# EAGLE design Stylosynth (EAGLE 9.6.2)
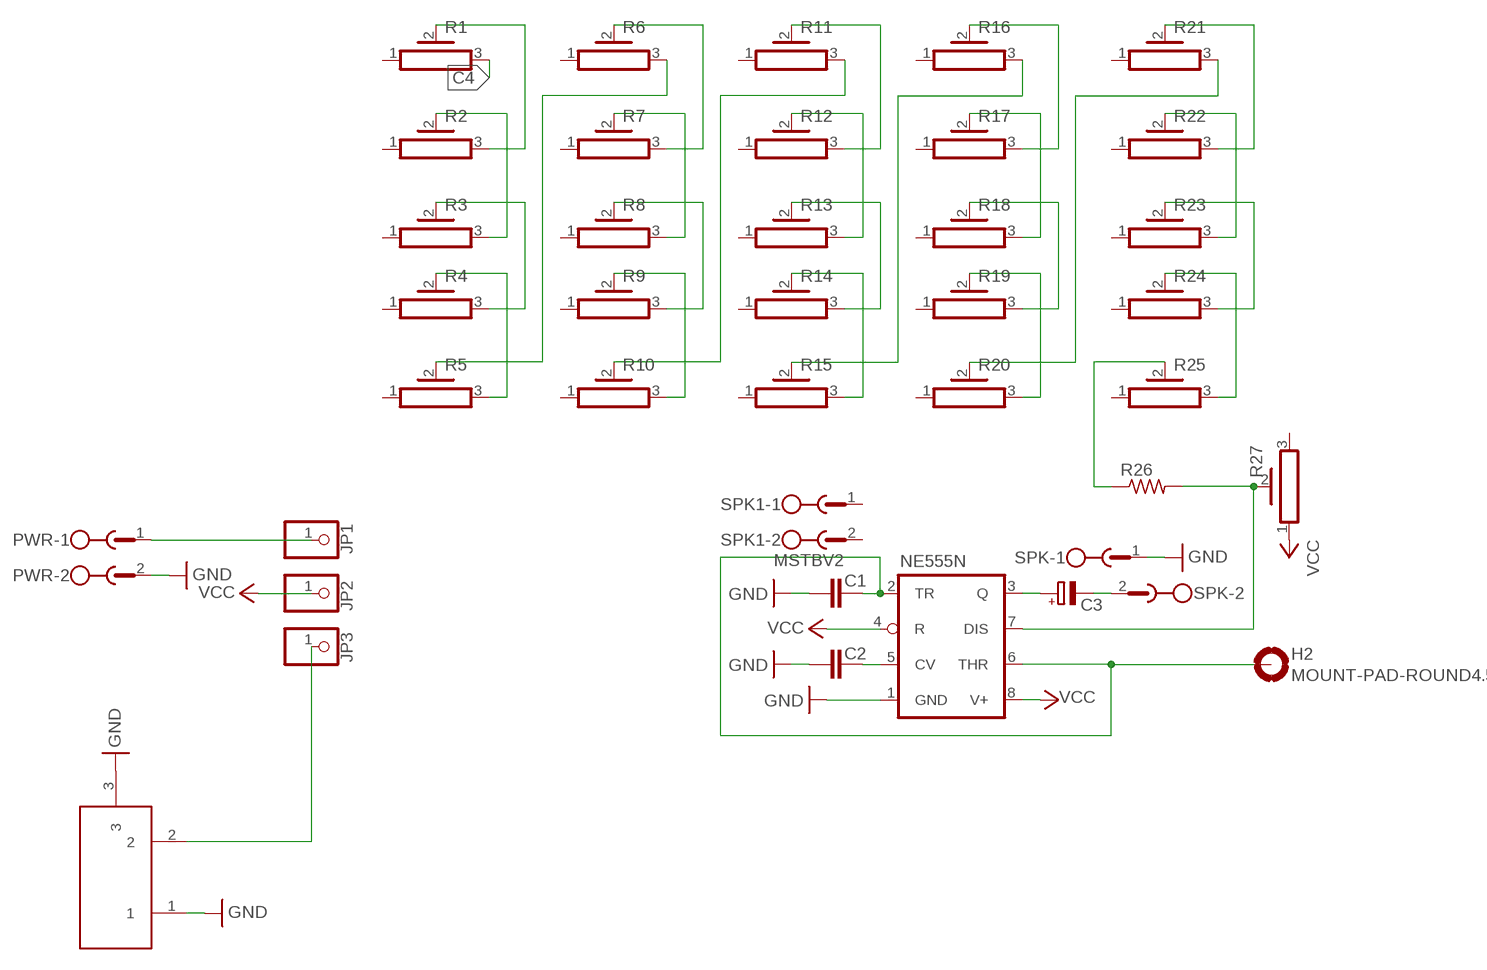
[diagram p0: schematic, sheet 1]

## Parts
C1  C5/2.5  [C5B2.5]
C2  C5/2.5  [C5B2.5]
C3  CPOL-EUE2.5-6  [E2,5-6]
H2  MOUNT-PAD-ROUND4.5  [4,5-PAD]
IC1  NE555N  [DIL08]
JP1  PINHD-1X01_2.54-90°  [1X01/90]
JP2  PINHD-1X01_2.54-90°  [1X01/90]
JP3  PINHD-1X01_2.54-90°  [1X01/90]
PWR  MSTBV2  [MSTBV2]
R1  POT_HA-06  [HA-06-SM065]
R2  POT_HA-06  [HA-06-SM065]
R3  POT_HA-06  [HA-06-SM065]
R4  POT_HA-06  [HA-06-SM065]
R5  POT_HA-06  [HA-06-SM065]
R6  POT_HA-06  [HA-06-SM065]
R7  POT_HA-06  [HA-06-SM065]
R8  POT_HA-06  [HA-06-SM065]
R9  POT_HA-06  [HA-06-SM065]
R10  POT_HA-06  [HA-06-SM065]
R11  POT_HA-06  [HA-06-SM065]
R12  POT_HA-06  [HA-06-SM065]
R13  POT_HA-06  [HA-06-SM065]
R14  POT_HA-06  [HA-06-SM065]
R15  POT_HA-06  [HA-06-SM065]
R16  POT_HA-06  [HA-06-SM065]
R17  POT_HA-06  [HA-06-SM065]
R18  POT_HA-06  [HA-06-SM065]
R19  POT_HA-06  [HA-06-SM065]
R20  POT_HA-06  [HA-06-SM065]
R21  POT_HA-06  [HA-06-SM065]
R22  POT_HA-06  [HA-06-SM065]
R23  POT_HA-06  [HA-06-SM065]
R24  POT_HA-06  [HA-06-SM065]
R25  POT_HA-06  [HA-06-SM065]
R26  R-US_0204/7  [0204/7]
R27  POT_HA-06  [HA-06-SM065]
SPK  MSTBV2  [MSTBV2]
SPK1  MSTBV2  [MSTBV2]
X1  DC21MMX  [DC-21MM]

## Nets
A4: R9.2 R10.3
A5: R21.2 R22.3
A#4: R10.2 R11.3
A#5: R22.2 R23.3
B4: R11.2 R12.3
B5: R23.2 R24.3
C4: R1.3
C5: R12.2 R13.3
C6: R24.2 R25.3
C#4: R1.2 R2.3
C#5: R13.2 R14.3
D4: R2.2 R3.3
D5: R14.2 R15.3
D#4: R3.2 R4.3
D#5: R15.2 R16.3
E4: R4.2 R5.3
E5: R16.2 R17.3
F4: R5.2 R6.3
F5: R17.2 R18.3
F#4: R6.2 R7.3
F#5: R18.2 R19.3
G4: R7.2 R8.3
G5: R19.2 R20.3
G#4: R8.2 R9.3
G#5: R20.2 R21.3
GND: C1.1 C2.1 IC1.1(GND) PWR.2 SPK.1 X1.1 X1.3
N$4: JP1.1 PWR.1
N$28: R25.2 R26.1
N$29: IC1.7(DIS) R26.2 R27.2
N$30: C3.+ IC1.3(Q)
N$31: C3.- SPK.2
N$32: C1.2 H2.B4,5(MOUNT) IC1.2(TR) IC1.6(THR)
N$33: C2.2 IC1.5(CV)
N$34: JP3.1 X1.2
VCC: IC1.4(R) IC1.8(V+) JP2.1 R27.1
Unconnected: R1.1 R2.1 R3.1 R4.1 R5.1 R6.1 R7.1 R8.1 R9.1 R10.1 R11.1 R12.1 R13.1 R14.1 R15.1 R16.1 R17.1 R18.1 R19.1 R20.1 R21.1 R22.1 R23.1 R24.1 R25.1 R27.3 SPK1.1 SPK1.2

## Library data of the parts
C1 C2 = capacitor-wima:C: CAPACITOR
C3 = rcl:CPOL-EU: POLARIZED CAPACITOR, European symbol; SPICEPREFIX: C
H2 = holes:MOUNT-PAD-ROUND: MOUNTING PAD, round
IC1 = linear:*555: TIMER
JP1-JP3 = pinhead-2:PINHD-1X01: PIN HEADER
PWR SPK SPK1 = con-phoenix-508:MSTBV2: PHOENIX; MPN: MSTBV 2,5/2-GF-5.08; OC_FARNELL: 1792792; OC_NEWARK: 69R9845
R1-R25 R27 = Tinkercad:POT: Rectangular Trimmer Potentiometers - PV36 Series Datasheet
R26 = rcl:R-US_: RESISTOR, American symbol; SPICEPREFIX: R
X1 = powersupply:DC21MM

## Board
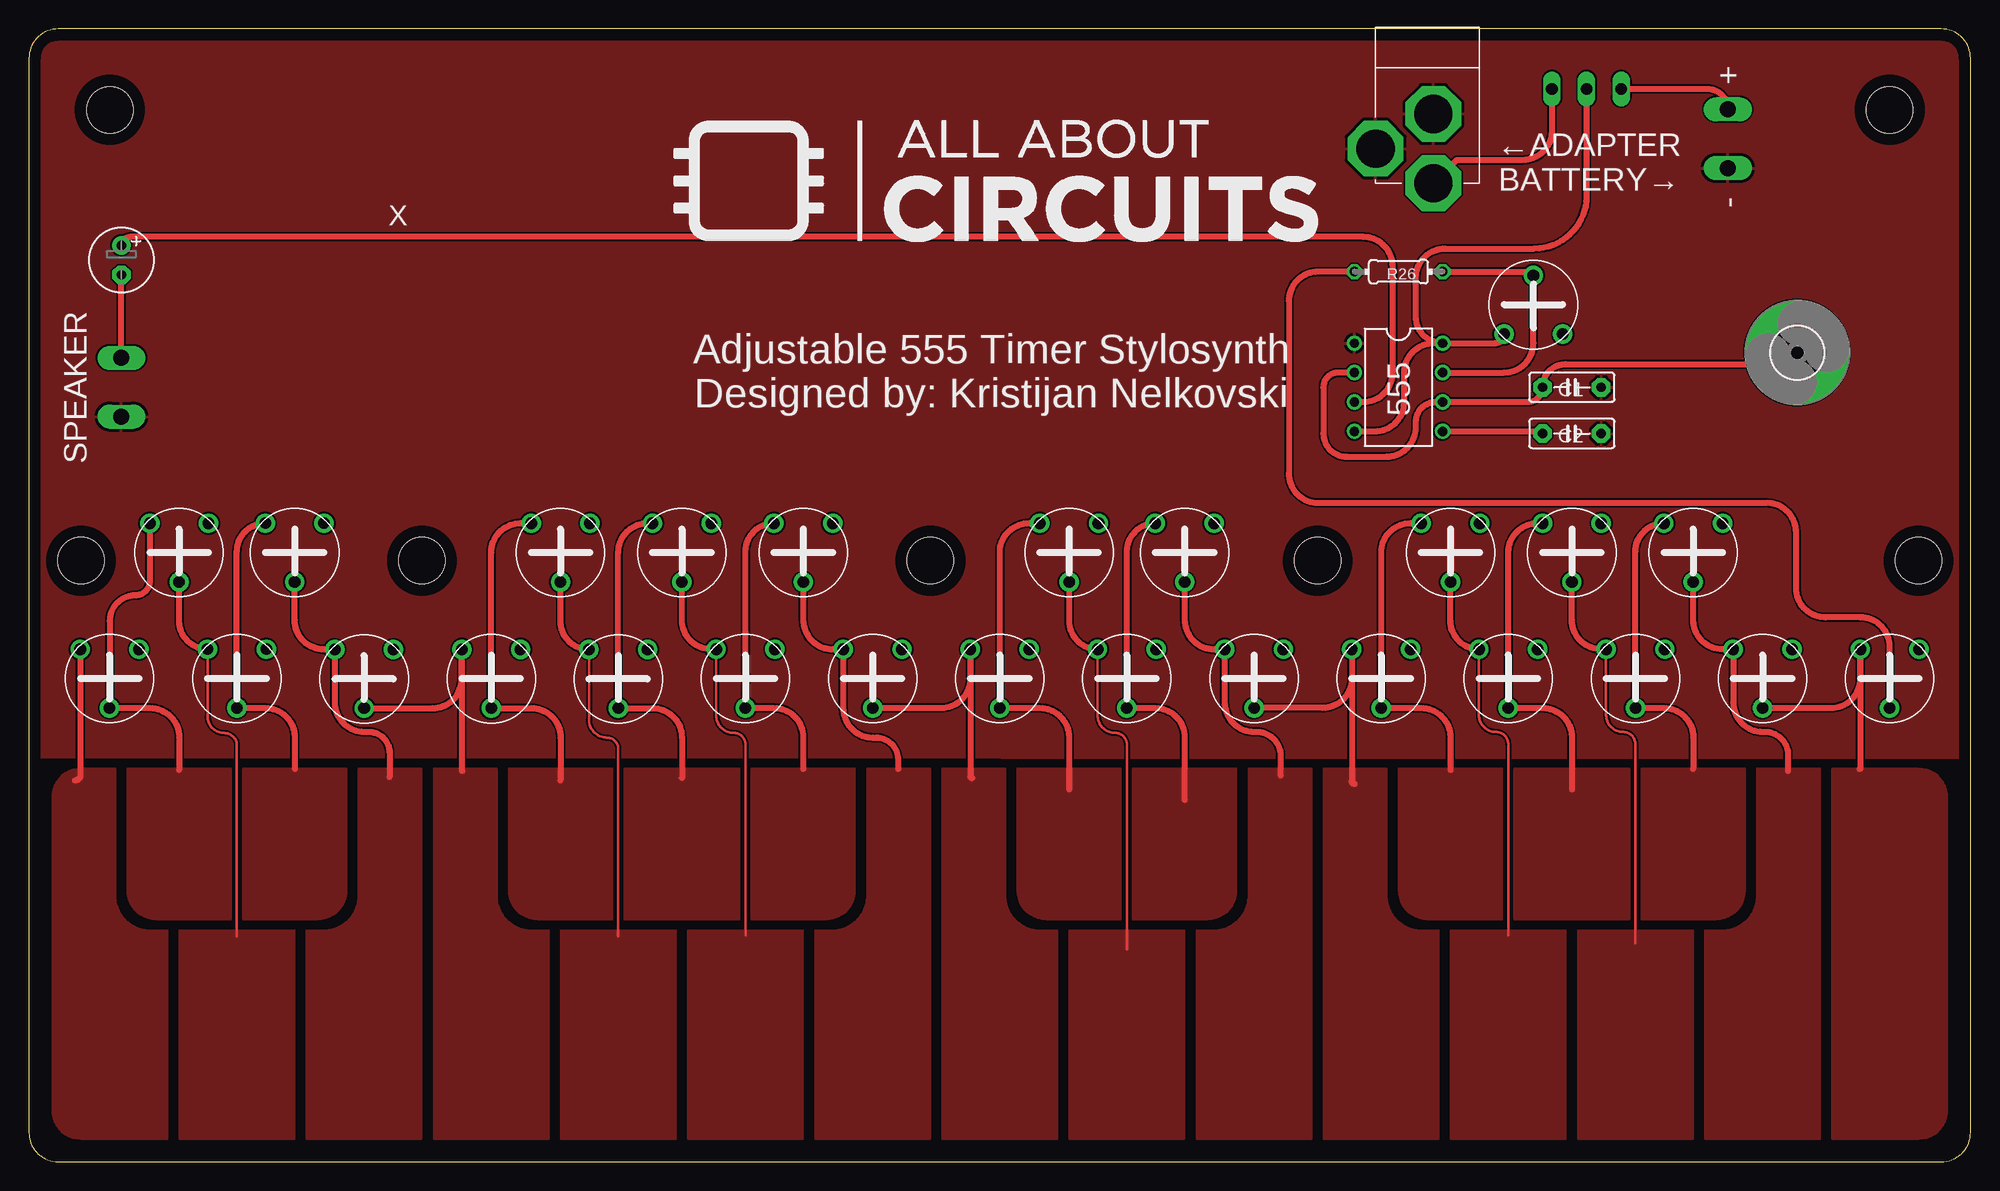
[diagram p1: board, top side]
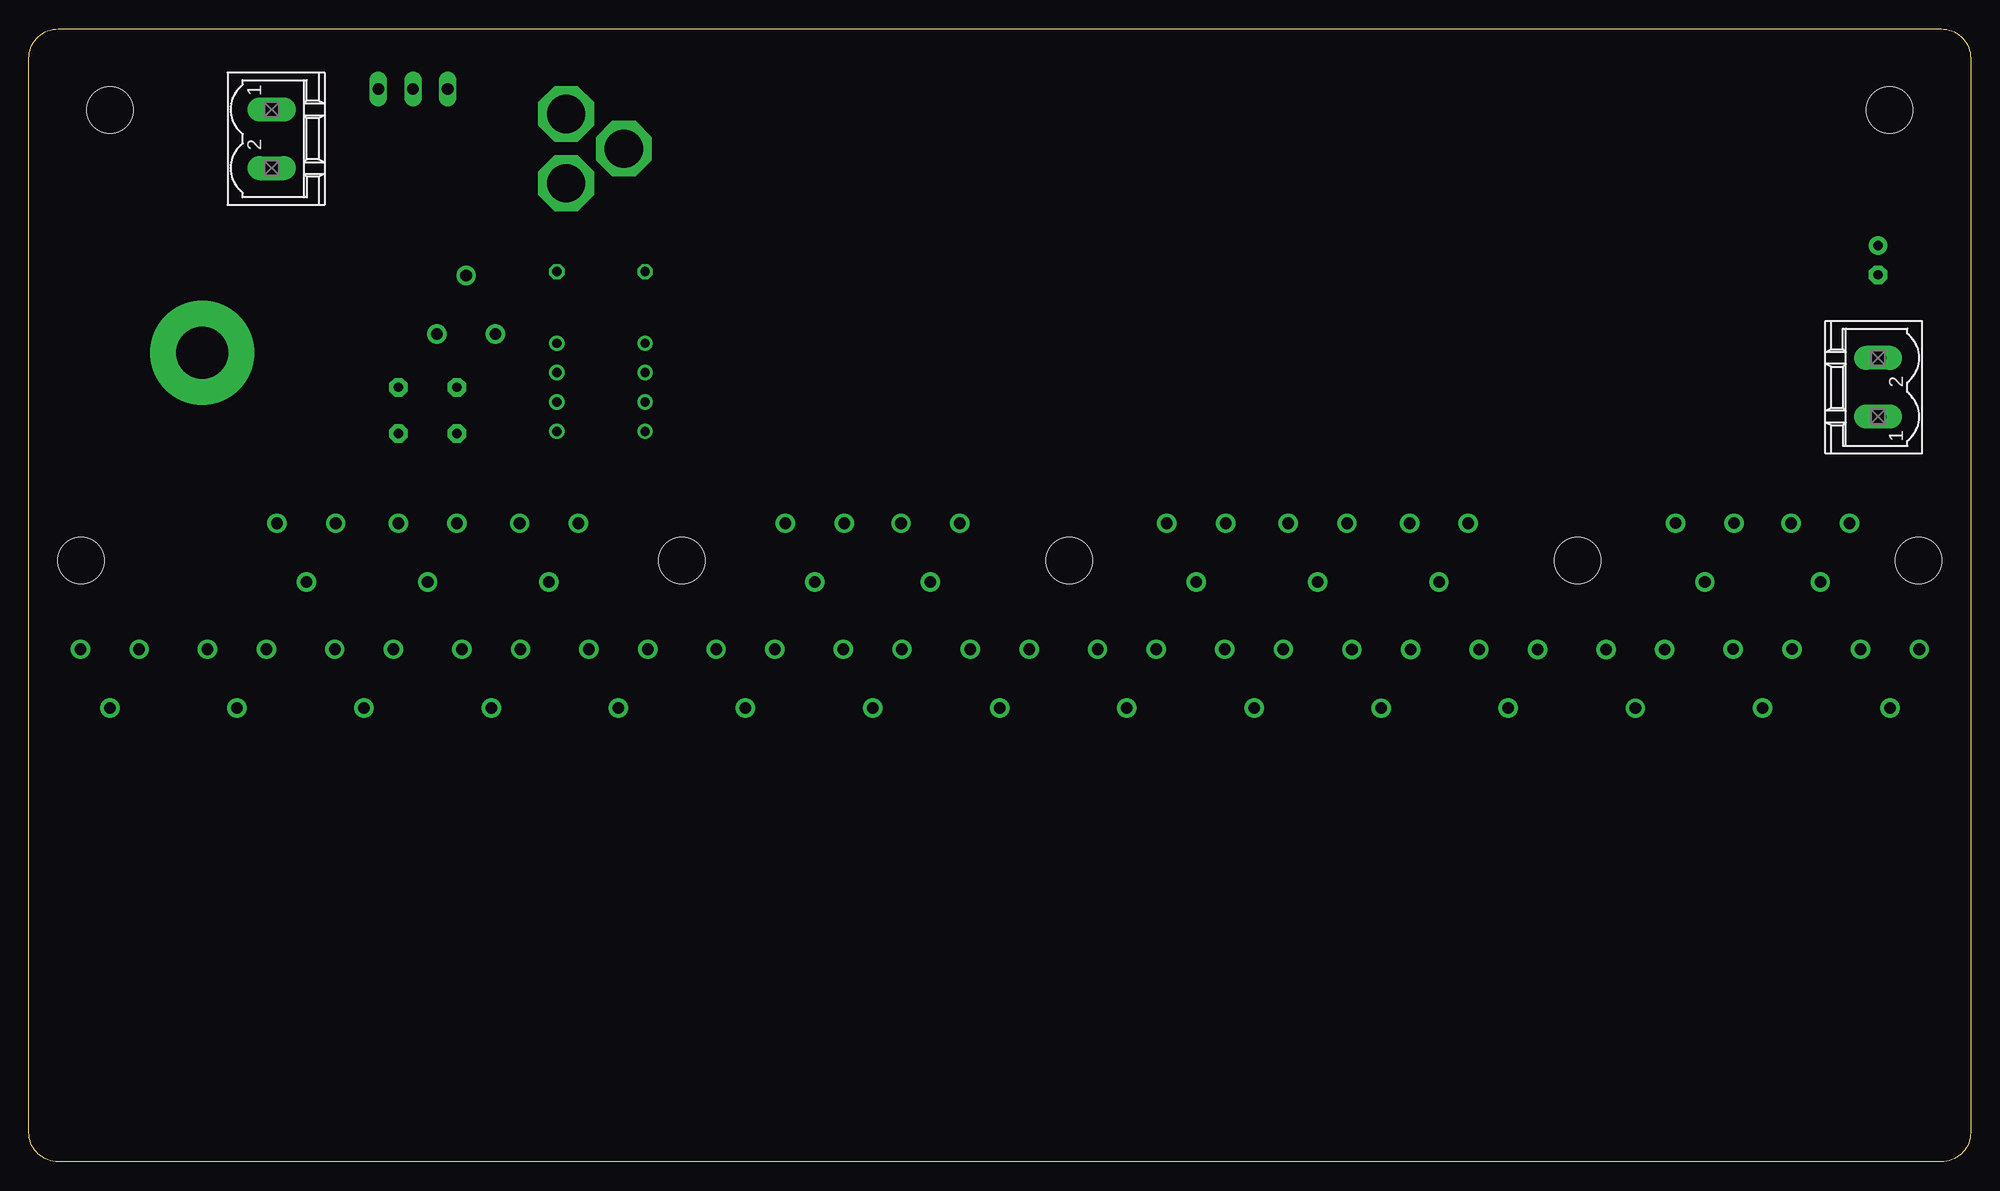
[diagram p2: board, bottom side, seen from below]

Size 168 x 98 mm. Coordinates in mm from the lower left corner, seen from the top.
Outline: 165.46,98 2.54,98 arc90 0,95.46 0,2.54 arc90 2.54,0 165.46,0 arc90 168,2.54 168,95.46 arc90 165.46,98
Copper layers (1*16): Top 0.035mm / dielectric 1.5mm / Bottom 0.035mm
Design rules "default": minimum track width 6mil, minimum drill 0.35mm, track to track 6mil, track to pad 6mil, pad to pad 6mil, via to via 6mil, smd to smd 6mil, copper to edge 40mil, drill to drill 6mil, minimum pad ring 10mil, minimum via ring 8mil, stop-mask expansion 4mil, vias tented up to drill 0mil, thermal gap 10mil
Holes 4 mm at 7,91 161,91 4.5,52 163.5,52 34,52 78,52 111.5,52

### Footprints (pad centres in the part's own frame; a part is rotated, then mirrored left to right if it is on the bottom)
C5B2.5 = drill 0.813 pad 1.6 octagon: 1 -2.54,0; 2 2.54,0
E2,5-6 = drill 0.813 pad 1.6: + -1.27,0 | drill 0.813 pad 1.6 octagon: - 1.27,0
4,5-PAD = drill 4.5 pad 9: B4,5 0,0
DIL08 = drill 0.813 pad 1.27: 1 -3.81,-3.81; 2 -1.27,-3.81; 3 1.27,-3.81; 4 3.81,-3.81; 5 3.81,3.81; 6 1.27,3.81; 7 -1.27,3.81; 8 -3.81,3.81
1X01/90 = drill 1.016 long: 1 -1.27,-3.81
MSTBV2 = drill 1.397 long: 1 -2.54,0; 2 2.54,0
HA-06-SM065 = drill 1 pad 1.676: 1 -2.54,-2.54; 2 0,2.54; 3 2.54,-2.54
0204/7 = drill 0.813 octagon: 1 -3.81,0; 2 3.81,0
DC-21MM = drill 3.302 pad 4.826 octagon: 1 -5.08,-3.353; 2 -0.076,-6.35; 3 -0.076,-0.356

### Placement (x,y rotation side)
C1  133.5,67 180 top
C2  133.5,63 180 top
C3  8,78 270 top
H2  153,70 0 top
IC1  118.5,67 270 top
JP1  136.5,89 180 top
JP2  133.5,89 180 top
JP3  130.5,89 180 top
PWR  147,88.5 270 bottom
R1  6.98,41.8 180 top
R2  13,52.7 180 top
R3  18,41.8 180 top
R4  23,52.7 180 top
R5  29.01,41.78 180 top
R6  40,41.79 180 top
R7  46,52.7 180 top
R8  50.99,41.78 180 top
R9  56.5,52.7 180 top
R10  62,41.8 180 top
R11  67,52.7 180 top
R12  73,41.8 180 top
R13  84,41.8 180 top
R14  90,52.7 180 top
R15  95,41.8 180 top
R16  100,52.7 180 top
R17  106,41.8 180 top
R18  117,41.8 180 top
R19  123,52.7 180 top
R20  128,41.8 180 top
R21  133.5,52.7 180 top
R22  139,41.8 180 top
R23  144,52.7 180 top
R24  150,41.8 180 top
R25  161,41.8 180 top
R26  118.5,77 0 top
R27  130.17,74.14 0 top
SPK  8,67 90 bottom
X1  121.6,91 0 top

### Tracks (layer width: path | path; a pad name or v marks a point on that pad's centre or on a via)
A4
  Top 0.2: R10.3 59.46,38.64 arc90 61,37.1 arc-90 62,36.1 62,19.6
  Top 0.5: R10.3 59.04,44.34 arc-90 56.5,46.88 R9.2
  pour Top: 57,2 67,2 67,20 57,20
A5
  Top 0.2: R22.3 136.46,38.64 arc90 137.9,37.2 arc-90 139,36.1 139,18.9
  Top 0.5: R22.3 136.04,44.34 arc-90 133.5,46.88 R21.2
  pour Top: 134,2 144,2 144,20 134,20
A#4
  Top 0.5: R11.3 arc90 62,52.78 R10.2 64.46,39.26 arc-90 67,36.72 67,34
  pour Top: 62.5,21 69,21 69.36,21.03 69.7,21.1 70.04,21.23 70.35,21.4 70.64,21.61 70.89,21.86 71.1,22.15 71.27,22.46 71.4,22.8 71.47,23.14 71.5,23.5 71.5,34 62.5,34
A#5
  Top 0.5: R23.3 arc90 139,52.78 R22.2 141.46,39.26 arc-90 144,36.72 144,34
  pour Top: 139.5,21 146,21 146.36,21.03 146.7,21.1 147.04,21.23 147.35,21.4 147.64,21.61 147.89,21.86 148.1,22.15 148.27,22.46 148.4,22.8 148.47,23.14 148.5,23.5 148.5,34 139.5,34
B4
  Top 0.5: R11.2 67,46.88 arc90 69.54,44.34 R12.3 70.46,39.24 arc90 73,36.7 73.3,36.7 arc-90 75.2,34.8 75.2,34
  pour Top: 68,2 78,2 78,34 72.5,34 72.5,23.02 72.5,23.01 72.5,23 72.5,22.99 72.5,22.98 72.47,22.59 72.47,22.58 72.47,22.57 72.47,22.56 72.47,22.56 72.38,22.17 72.38,22.16 72.38,22.15 72.38,22.15 72.37,22.14 72.23,21.77 72.23,21.76 72.23,21.75 72.23,21.74 72.22,21.74 72.03,21.39 72.03,21.39 72.02,21.38 72.02,21.37 72.01,21.37 71.78,21.05 71.77,21.04 71.77,21.04 71.76,21.03 71.76,21.02 71.48,20.74 71.47,20.74 71.46,20.73 71.46,20.73 71.45,20.72 71.13,20.49 71.13,20.48 71.12,20.48 71.11,20.47 71.11,20.47 70.76,20.28 70.76,20.27 70.75,20.27 70.74,20.27 70.73,20.27 70.36,20.13 70.35,20.12 70.35,20.12 70.34,20.12 70.33,20.12 69.94,20.03 69.94,20.03 69.93,20.03 69.92,20.03 69.91,20.03 69.52,20 69.51,20 69.5,20 69.49,20 69.48,20 68,20
B5
  Top 0.5: R23.2 144,46.88 arc90 146.54,44.34 R24.3 147.46,39.74 arc90 150,37.2 150.2,37.2 arc-90 152.2,35.2 152.2,33.8
  pour Top: 145,2 155,2 155,34 149.5,34 149.5,23.02 149.5,23.01 149.5,23 149.5,22.99 149.5,22.98 149.47,22.59 149.47,22.58 149.47,22.57 149.47,22.56 149.47,22.56 149.38,22.17 149.38,22.16 149.38,22.15 149.38,22.15 149.37,22.14 149.23,21.77 149.23,21.76 149.23,21.75 149.23,21.74 149.22,21.74 149.03,21.39 149.03,21.39 149.02,21.38 149.02,21.37 149.01,21.37 148.78,21.05 148.77,21.04 148.77,21.04 148.76,21.03 148.76,21.02 148.48,20.74 148.47,20.74 148.46,20.73 148.46,20.73 148.45,20.72 148.13,20.49 148.13,20.48 148.12,20.48 148.11,20.47 148.11,20.47 147.76,20.28 147.76,20.27 147.75,20.27 147.74,20.27 147.73,20.27 147.36,20.13 147.35,20.12 147.35,20.12 147.34,20.12 147.33,20.12 146.94,20.03 146.94,20.03 146.93,20.03 146.92,20.03 146.91,20.03 146.52,20 146.51,20 146.5,20 146.49,20 146.48,20 145,20
C4
  Top 0.5: 4,33 arc90 4.46,33.46 arc-90 4.44,33.48 4.44,33.9 R1.3
  pour Top: 4.5,2 12,2 12,20 10.52,20 10.51,20 10.5,20 10.49,20 10.48,20 10.09,20.03 10.08,20.03 10.07,20.03 10.06,20.03 10.06,20.03 9.67,20.12 9.66,20.12 9.65,20.12 9.65,20.12 9.64,20.13 9.27,20.27 9.26,20.27 9.25,20.27 9.24,20.27 9.24,20.28 8.89,20.47 8.89,20.47 8.88,20.48 8.87,20.48 8.87,20.49 8.55,20.72 8.54,20.73 8.54,20.73 8.53,20.74 8.52,20.74 8.24,21.02 8.24,21.03 8.23,21.04 8.23,21.04 8.22,21.05 7.99,21.37 7.98,21.37 7.98,21.38 7.97,21.39 7.97,21.39 7.78,21.74 7.77,21.74 7.77,21.75 7.77,21.76 7.77,21.77 7.63,22.14 7.62,22.15 7.62,22.15 7.62,22.16 7.62,22.17 7.53,22.56 7.53,22.56 7.53,22.57 7.53,22.58 7.53,22.59 7.5,22.98 7.5,22.99 7.5,23 7.5,23.01 7.5,23.02 7.5,34 4.5,34 4.14,33.97 3.8,33.9 3.46,33.77 3.15,33.6 2.86,33.39 2.61,33.14 2.4,32.85 2.23,32.54 2.1,32.2 2.03,31.86 2,31.5 2,4.5 2.03,4.14 2.1,3.8 2.23,3.46 2.4,3.15 2.61,2.86 2.86,2.61 3.15,2.4 3.46,2.23 3.8,2.1 4.14,2.03
C5
  Top 0.5: R12.2 78.92,39.26 arc90 81.46,41.8 R13.3 81.46,33.34 arc90 81.6,33.2
  pour Top: 79,2 89,2 89,20 87.52,20 87.51,20 87.5,20 87.49,20 87.48,20 87.09,20.03 87.08,20.03 87.07,20.03 87.06,20.03 87.06,20.03 86.67,20.12 86.66,20.12 86.65,20.12 86.65,20.12 86.64,20.13 86.27,20.27 86.26,20.27 86.25,20.27 86.24,20.27 86.24,20.28 85.89,20.47 85.89,20.47 85.88,20.48 85.87,20.48 85.87,20.49 85.55,20.72 85.54,20.73 85.54,20.73 85.53,20.74 85.52,20.74 85.24,21.02 85.24,21.03 85.23,21.04 85.23,21.04 85.22,21.05 84.99,21.37 84.98,21.37 84.98,21.38 84.97,21.39 84.97,21.39 84.78,21.74 84.77,21.74 84.77,21.75 84.77,21.76 84.77,21.77 84.63,22.14 84.62,22.15 84.62,22.15 84.62,22.16 84.62,22.17 84.53,22.56 84.53,22.56 84.53,22.57 84.53,22.58 84.53,22.59 84.5,22.98 84.5,22.99 84.5,23 84.5,23.01 84.5,23.02 84.5,34 79,34
C6
  Top 0.5: R24.2 155.92,39.26 arc90 158.46,41.8 R25.3 158.46,34.06 arc-90 158.4,34
  pour Top: 156,2 163.5,2 163.86,2.03 164.2,2.1 164.54,2.23 164.85,2.4 165.14,2.61 165.39,2.86 165.6,3.15 165.77,3.46 165.9,3.8 165.97,4.14 166,4.5 166,31.5 165.97,31.86 165.9,32.2 165.77,32.54 165.6,32.85 165.39,33.14 165.14,33.39 164.85,33.6 164.54,33.77 164.2,33.9 163.86,33.97 163.5,34 156,34
C#4
  Top 0.5: R2.3 10.46,50.26 arc-90 9.2,49 arc90 6.98,46.78 R1.2 10.46,39.26 arc-90 13,36.72 13,33.9
  pour Top: 11,21 17.5,21 17.5,34 8.5,34 8.5,23.5 8.53,23.14 8.6,22.8 8.73,22.46 8.9,22.15 9.11,21.86 9.36,21.61 9.65,21.4 9.96,21.23 10.3,21.1 10.64,21.03
C#5
  Top 0.5: R14.3 86.54,55.24 arc90 84,52.7 R13.2 87.46,39.26 arc-90 90,36.72 90,32.2
  pour Top: 88,21 94.5,21 94.5,34 85.5,34 85.5,23.5 85.53,23.14 85.6,22.8 85.73,22.46 85.9,22.15 86.11,21.86 86.36,21.61 86.65,21.4 86.96,21.23 87.3,21.1 87.64,21.03
D4
  Top 0.2: R3.3 15.46,38.54 arc90 16.9,37.1 arc-90 18,36 18,19.5
  Top 0.5: R3.3 arc-90 13,46.8 R2.2
  pour Top: 13,2 23,2 23,20 13,20
D5
  Top 0.2: R15.3 92.46,38.64 arc90 94,37.1 arc-90 95,36.1 95,18.4
  Top 0.5: R14.2 90,46.8 arc90 R15.3
  pour Top: 90,2 100,2 100,20 90,20
D#4
  Top 0.5: 23,34 23,36.72 arc90 20.46,39.26 R3.2 18,52.78 arc-90 R4.3
  pour Top: 18.5,21 25,21 25.36,21.03 25.7,21.1 26.04,21.23 26.35,21.4 26.64,21.61 26.89,21.86 27.1,22.15 27.27,22.46 27.4,22.8 27.47,23.14 27.5,23.5 27.5,34 18.5,34
D#5
  Top 0.5: R16.3 arc90 95,52.78 R15.2 97.46,39.26 arc-90 100,36.72 100,31.3
  pour Top: 95.5,21 102,21 102.36,21.03 102.7,21.1 103.04,21.23 103.35,21.4 103.64,21.61 103.89,21.86 104.1,22.15 104.27,22.46 104.4,22.8 104.47,23.14 104.5,23.5 104.5,34 95.5,34
E4
  Top 0.5: R4.2 23,46.86 arc90 25.54,44.32 R5.3 26.47,39.74 arc90 29.01,37.2 29.4,37.2 arc-90 31.2,35.4 31.2,33.3
  pour Top: 24,2 34,2 34,34 28.5,34 28.5,23.02 28.5,23.01 28.5,23 28.5,22.99 28.5,22.98 28.47,22.59 28.47,22.58 28.47,22.57 28.47,22.56 28.47,22.56 28.38,22.17 28.38,22.16 28.38,22.15 28.38,22.15 28.37,22.14 28.23,21.77 28.23,21.76 28.23,21.75 28.23,21.74 28.22,21.74 28.03,21.39 28.03,21.39 28.02,21.38 28.02,21.37 28.01,21.37 27.78,21.05 27.77,21.04 27.77,21.04 27.76,21.03 27.76,21.02 27.48,20.74 27.47,20.74 27.46,20.73 27.46,20.73 27.45,20.72 27.13,20.49 27.13,20.48 27.12,20.48 27.11,20.47 27.11,20.47 26.76,20.28 26.76,20.27 26.75,20.27 26.74,20.27 26.73,20.27 26.36,20.13 26.35,20.12 26.35,20.12 26.34,20.12 26.33,20.12 25.94,20.03 25.94,20.03 25.93,20.03 25.92,20.03 25.91,20.03 25.52,20 25.51,20 25.5,20 25.49,20 25.48,20 24,20
E5
  Top 0.5: R16.2 100,46.88 arc90 102.54,44.34 R17.3 103.46,39.74 arc90 106,37.2 106.2,37.2 arc-90 108.3,35.1 108.3,33.4
  pour Top: 101,2 111,2 111,34 105.5,34 105.5,23.02 105.5,23.01 105.5,23 105.5,22.99 105.5,22.98 105.47,22.59 105.47,22.58 105.47,22.57 105.47,22.56 105.47,22.56 105.38,22.17 105.38,22.16 105.38,22.15 105.38,22.15 105.37,22.14 105.23,21.77 105.23,21.76 105.23,21.75 105.23,21.74 105.22,21.74 105.03,21.39 105.03,21.39 105.02,21.38 105.02,21.37 105.01,21.37 104.78,21.05 104.77,21.04 104.77,21.04 104.76,21.03 104.76,21.02 104.48,20.74 104.47,20.74 104.46,20.73 104.46,20.73 104.45,20.72 104.13,20.49 104.13,20.48 104.12,20.48 104.11,20.47 104.11,20.47 103.76,20.28 103.76,20.27 103.75,20.27 103.74,20.27 103.73,20.27 103.36,20.13 103.35,20.12 103.35,20.12 103.34,20.12 103.33,20.12 102.94,20.03 102.94,20.03 102.93,20.03 102.92,20.03 102.91,20.03 102.52,20 102.51,20 102.5,20 102.49,20 102.48,20 101,20
F4
  Top 0.5: R5.2 34.92,39.24 arc90 37.46,41.78 R6.3 37.46,33.84 arc90 37.5,33.8
  pour Top: 35,2 45,2 45,20 43.52,20 43.51,20 43.5,20 43.49,20 43.48,20 43.09,20.03 43.08,20.03 43.07,20.03 43.06,20.03 43.06,20.03 42.67,20.12 42.66,20.12 42.65,20.12 42.65,20.12 42.64,20.13 42.27,20.27 42.26,20.27 42.25,20.27 42.24,20.27 42.24,20.28 41.89,20.47 41.89,20.47 41.88,20.48 41.87,20.48 41.87,20.49 41.55,20.72 41.54,20.73 41.54,20.73 41.53,20.74 41.52,20.74 41.24,21.02 41.24,21.03 41.23,21.04 41.23,21.04 41.22,21.05 40.99,21.37 40.98,21.37 40.98,21.38 40.97,21.39 40.97,21.39 40.78,21.74 40.77,21.74 40.77,21.75 40.77,21.76 40.77,21.77 40.63,22.14 40.62,22.15 40.62,22.15 40.62,22.16 40.62,22.17 40.53,22.56 40.53,22.56 40.53,22.57 40.53,22.58 40.53,22.59 40.5,22.98 40.5,22.99 40.5,23 40.5,23.01 40.5,23.02 40.5,34 35,34
F5
  Top 0.5: R17.2 111.92,39.26 arc90 114.46,41.8 R18.3 114.46,32.94 arc90 114.7,32.7
  pour Top: 112,2 122,2 122,20 120.52,20 120.51,20 120.5,20 120.49,20 120.48,20 120.09,20.03 120.08,20.03 120.07,20.03 120.06,20.03 120.06,20.03 119.67,20.12 119.66,20.12 119.65,20.12 119.65,20.12 119.64,20.13 119.27,20.27 119.26,20.27 119.25,20.27 119.24,20.27 119.24,20.28 118.89,20.47 118.89,20.47 118.88,20.48 118.87,20.48 118.87,20.49 118.55,20.72 118.54,20.73 118.54,20.73 118.53,20.74 118.52,20.74 118.24,21.02 118.24,21.03 118.23,21.04 118.23,21.04 118.22,21.05 117.99,21.37 117.98,21.37 117.98,21.38 117.97,21.39 117.97,21.39 117.78,21.74 117.77,21.74 117.77,21.75 117.77,21.76 117.77,21.77 117.63,22.14 117.62,22.15 117.62,22.15 117.62,22.16 117.62,22.17 117.53,22.56 117.53,22.56 117.53,22.57 117.53,22.58 117.53,22.59 117.5,22.98 117.5,22.99 117.5,23 117.5,23.01 117.5,23.02 117.5,34 112,34
F#4
  Top 0.5: R7.3 42.54,55.24 arc90 40,52.7 R6.2 43.46,39.25 arc-90 46,36.71 46,33
  pour Top: 44,21 50.5,21 50.5,34 41.5,34 41.5,23.5 41.53,23.14 41.6,22.8 41.73,22.46 41.9,22.15 42.11,21.86 42.36,21.61 42.65,21.4 42.96,21.23 43.3,21.1 43.64,21.03
F#5
  Top 0.5: R19.3 119.54,55.24 arc90 117,52.7 R18.2 120.46,39.26 arc-90 123,36.72 123,33.9
  pour Top: 121,21 127.5,21 127.5,34 118.5,34 118.5,23.5 118.53,23.14 118.6,22.8 118.73,22.46 118.9,22.15 119.11,21.86 119.36,21.61 119.65,21.4 119.96,21.23 120.3,21.1 120.64,21.03
G4
  Top 0.2: R8.3 48.45,38.25 arc90 50,36.7 arc-90 51,35.7 51,19.6 51,19.5
  Top 0.5: R8.3 arc-90 46,46.77 R7.2
  pour Top: 46,2 56,2 56,20 46,20
G5
  Top 0.2: R20.3 125.46,38.64 arc90 126.9,37.2 arc-90 128,36.1 128,19.6
  Top 0.5: R20.3 arc-90 123,46.8 R19.2
  pour Top: 123,2 133,2 133,20 123,20
G#4
  Top 0.5: R9.3 53.53,55.24 arc90 50.99,52.7 R8.2 53.96,39.24 arc-90 56.5,36.7 56.5,33.2
  pour Top: 51.5,21 61.5,21 61.5,34 51.5,34
G#5
  Top 0.5: R21.3 130.54,55.24 arc90 128,52.7 R20.2 130.96,39.26 arc-90 133.5,36.72 133.5,32.2
  pour Top: 128.5,21 138.5,21 138.5,34 128.5,34
GND
  Top 0.5: IC1.1 114.54,70.81
  pour Top: 168.2,34.9 168.2,98 0,98 0,35
N$4
  Top 0.5: JP1.1 145.23,92.81 arc-90 PWR.1
N$28
  Top 0.5: R26.1 111.54,77 arc90 109,74.46 109,59.54 arc90 111.54,57 150.36,57 arc-90 152.9,54.46 152.9,49.64 arc90 155.44,47.1 158.46,47.1 arc-90 161,44.56 R25.2
N$29
  Top 0.5: R26.2 129.85,77 arc-90 R27.2 130.17,70.81 arc-90 127.63,68.27 IC1.7
N$30
  Top 0.5: IC1.3 115.46,65.73 arc90 118,68.27 118,77.46 arc90 115.46,80 8.73,80 arc90 C3.+
N$31
  Top 0.5: SPK.2 C3.-
N$32
  Top 0.5: H2.B4,5 153,69 132.96,69 arc90 C1.2 arc-90 129.69,65.73 IC1.6 121.73,65.73 arc90 120,64 120,63.54 arc-90 117.46,61 114,61 arc-90 112,63 112,67 arc-90 113.27,68.27 IC1.2
N$33
  Top 0.5: IC1.5 130.77,63.19 arc-90 C2.2
N$34
  Top 0.5: JP3.1 131.77,89.19 arc-90 129.23,86.65 123.52,86.65 X1.2
VCC
  Top 0.5: JP2.1 134.77,83.54 arc-90 130.23,79 122.54,79 arc90 120,76.46 120,73.12 arc90 IC1.8 | IC1.8 121.54,70.81 arc90 119,68.27 119,65.73 arc-90 116.46,63.19 IC1.4 | IC1.8 126.84,70.81 arc90 R27.1
(copper drawn outside any net)
  shapes: Top area x2

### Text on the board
tPlace: + | ←ADAPTER | BATTERY→ | - | X | Adjustable 555 Timer Stylosynth / Designed by: Kristijan Nelkovski | SPEAKER | 555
